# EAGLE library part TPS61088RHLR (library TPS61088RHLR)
10-A Fully-Integrated Synchronous Boost Converter Source: Datasheet
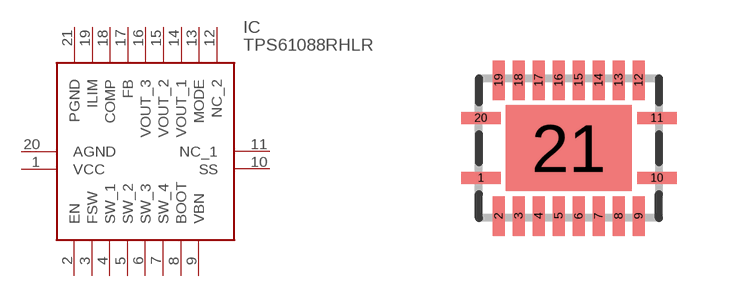
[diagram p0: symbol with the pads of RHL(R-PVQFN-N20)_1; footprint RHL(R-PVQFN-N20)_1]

Designator prefix IC

## TPS61088RHLR (Arrow_Part_Number: TPS61088RHLR; Arrow_Price-Stock: https://www.arrow.com/en/products/tps61088rhlr/texas-instruments?utm_currency=USD&region=nac; Description: 10-A Fully-Integrated Synchronous Boost Converter; Height: mm; Manufacturer_Name: Texas Instruments; Manufacturer_Part_Number: TPS61088RHLR; Mouser_Part_Number: 595-TPS61088RHLR; Mouser_Price-Stock: https://www.mouser.co.uk/ProductDetail/Texas-Instruments/TPS61088RHLR?qs=MiqG6Kq1qKNjgpnslrNKug%3D%3D)  [RHL(R-PVQFN-N20)_1]
1  VCC
2  EN
3  FSW
4  SW_1
5  SW_2
6  SW_3
7  SW_4
8  BOOT
9  VBN
10  SS
11  NC_1
12  NC_2
13  MODE
14  VOUT_1
15  VOUT_2
16  VOUT_3
17  FB
18  COMP
19  ILIM
20  AGND
21  PGND

## Footprint RHL(R-PVQFN-N20)_1 (pad centres in mm)
RHL(R-PVQFN-N20)_1
smd 0.99 x 0.3: 1 -2.2,-0.75; 10 2.2,-0.75; 11 2.2,0.75; 20 -2.2,0.75
smd 0.3 x 0.99: 2 -1.75,-1.7; 3 -1.25,-1.7; 4 -0.75,-1.7; 5 -0.25,-1.7; 6 0.25,-1.7; 7 0.75,-1.7; 8 1.25,-1.7; 9 1.75,-1.7; 12 1.75,1.7; 13 1.25,1.7; 14 0.75,1.7; 15 0.25,1.7; 16 -0.25,1.7; 17 -0.75,1.7; 18 -1.25,1.7; 19 -1.75,1.7
smd 3.15 x 2.15: 21 0,0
